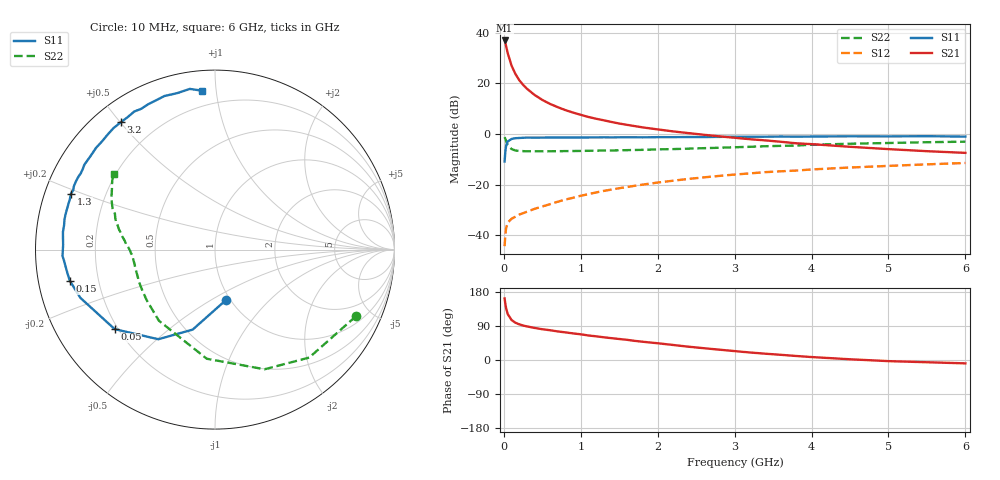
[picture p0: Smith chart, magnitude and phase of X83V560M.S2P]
! SIEMENS Small Signal Semiconductors
! BFP136W
! Si NPN RF Bipolar Junction Transistor in SOT343
! VCE = 3.5 V  IC = 60 mA
! Common Emitter S-Parameters:  September  1994
# GHz  S  MA  R  50
!  f  S11  S21  S12  S22
! GHz  MAG  ANG  MAG  ANG  MAG  ANG  MAG  ANG
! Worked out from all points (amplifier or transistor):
!   40 points, 10 MHz to 6 GHz, reference 50 ohm
!   highest |S21| = 36.9 dB at 10 MHz (marker M1)
!   |S21| within 3 dB of that: start of sweep to 35.16 MHz
!   unconditionally stable (mu >= 1): 635.3 MHz to 2.868 GHz
!   at 200 MHz: K = 0.58, MSG = 26.6 dB, |S12| = -31.8 dB
!   at 1.5 GHz: K = 1.10, MAG = 10.9 dB, |S12| = -21.4 dB
!   at 6 GHz: K = 0.97, MSG = 2.0 dB, |S12| = -11.4 dB
!   S11 on the Smith chart (normalised r, x): 10 MHz: 0.96, -0.58; 50 MHz: 0.19, -0.34; 150 MHz: 0.10, -0.11; 1.3 GHz: 0.08, +0.19; 3.2 GHz: 0.08, +0.50; 6 GHz: 0.11, +0.92
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0.01  0.2866 -77.4  70.35 162.5  0.0061 73.0  0.8687 -25.3
0.02  0.4628 -105.6  62.04 147.4  0.0105 60.5  0.7984 -48.9
0.03  0.5908 -122.3  53.88 136.1  0.014 51.6  0.7217 -67.5
0.05  0.7133 -141.6  39.72 121.4  0.0177 40.7  0.6099 -94.3
0.1  0.7968 -160.3  22.49 105.6  0.0212 33.5  0.5046 -128.3
0.15  0.8274 -167.9  15.39 98.4  0.0233 34.3  0.4732 -143.7
0.2  0.835 -172.1  11.59 94.2  0.0256 36.2  0.4632 -152.2
0.25  0.8421 -175.4  9.364 91.0  0.0273 38.3  0.4594 -157.7
0.3  0.8504 -177.6  7.839 88.7  0.0292 41.0  0.4558 -161.3
0.4  0.8465 178.3  5.904 84.6  0.0333 44.8  0.4556 -166.2
0.5  0.8496 175.5  4.71 81.2  0.0371 48.3  0.4556 -169.4
0.6  0.8529 173.3  3.931 78.6  0.0411 50.5  0.4567 -171.4
0.7  0.8517 170.8  3.39 75.4  0.046 53.3  0.4584 -172.9
0.9  0.8555 167.0  2.65 70.2  0.0551 55.6  0.4613 -175.5
1.1  0.8554 162.5  2.168 64.7  0.065 57.2  0.4661 -177.1
1.3  0.8609 158.8  1.863 59.9  0.0753 57.8  0.4714 -178.7
1.7  0.8625 151.8  1.434 50.5  0.0949 56.9  0.4837 178.4
2.2  0.8672 143.4  1.126 39.7  0.1197 54.2  0.5036 174.8
3.2  0.8825 126.4  0.789 19.8  0.167 45.9  0.5589 166.0
4.5  0.9009 108.2  0.559 1.9  0.218 34.0  0.6432 153.8
5.5  0.9063 98.9  0.458 -5.9  0.2516 26.2  0.6886 146.3
6  0.8879 94.6  0.424 -8.9  0.2681 21.8  0.706 143.1
